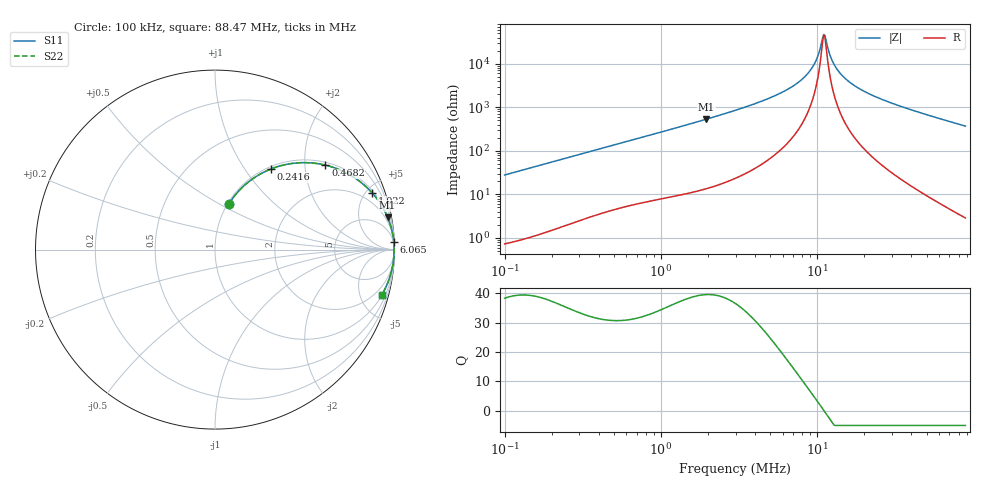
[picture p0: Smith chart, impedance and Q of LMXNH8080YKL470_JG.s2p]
! LMXNH8080YKL470_JG  S-PARAMETER MODEL  ( General Type )
! Model Generated by TAIYO YUDEN Corporation (http://www.ty-top.com)
! Version 1.0
! TAIYO YUDEN Control No. 191025NI43SB-FBB
! Copyright(c) 2019 TAIYO YUDEN CO.,LTD. All Rights Reserved.
! Product Description (link to TY-COMPAS)
! https://ds.yuden.co.jp/TYCOMPAS/or/detail?pn=LMXNH8080YKL470MJG&u=M
! Products Name : Inductors
! Characteristics :
!  Inductance : 47 uH , SRF(min) : 8.0 MHz , DC Resistance(max) : 0.182 Ohm
!  Rated Current : Saturation :1500 mA , Temp Rise : 1500 mA
!  Case Size : 8.0 x 8.0 / 0.315 x 0.315 [mm/inch] , Thickness : 4 / 0.157 [mm/inch]
!  (Conditions: Temperature = 25 degC , DC Bias Current/Voltage = 0A / 0V)
! External Node Assignments :
!  1  o---GGG---o  2
! GND o---------o GND
! Frequency Range : 0.1MHz  -  88.465963MHz  [ 402 STEP ]
# MHz S RI R 50
! Freq[MHz].  S11 Real  S11 Imag  S21 Real  S21 Imag  S12 Real  S12 Imag  S22 Real  S22 Imag
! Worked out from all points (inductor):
!   401 points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, 100 kHz to 88.47 MHz, reference 50 ohm
!   read as one part in series: L = 44.1 uH near 103.5 kHz
!   highest Q = 39.5 at 1.946 MHz (marker M1), where L = 43.4 uH
!   self-resonance near 10.98 MHz
!   S11 on the Smith chart (normalised r, x): 100 kHz: 1.01, +0.56; 241.6 kHz: 1.04, +1.33; 468.2 kHz: 1.08, +2.54; 1.022 MHz: 1.16, +5.49; 6.065 MHz: 3, +46; 88.47 MHz: 1.06, -7.38
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0.1  0.0774 0.2545  0.9226 -0.2545  0.9226 -0.2545  0.0774 0.2545
0.155432  0.1627 0.3565  0.8373 -0.3565  0.8373 -0.3565  0.1627 0.3565
0.241591  0.312 0.4494  0.688 -0.4494  0.688 -0.4494  0.312 0.4494
0.311591  0.4245 0.4794  0.5755 -0.4794  0.5755 -0.4794  0.4245 0.4794
0.468157  0.6148 0.4707  0.3852 -0.4707  0.3852 -0.4707  0.6148 0.4707
0.97089  0.8648 0.3276  0.1352 -0.3276  0.1352 -0.3276  0.8648 0.3276
1.021576  0.8759 0.3156  0.1241 -0.3156  0.1241 -0.3156  0.8759 0.3156
1.946322  0.9615 0.1801  0.0385 -0.1801  0.0385 -0.1801  0.9615 0.1801
2.974323  0.9832 0.1158  0.0168 -0.1158  0.0168 -0.1158  0.9832 0.1158
6.064564  0.9958 0.0434  0.00419 -0.0434  0.00419 -0.0434  0.9958 0.0434
7.821746  0.9972 0.024  0.00276 -0.024  0.00276 -0.024  0.9972 0.024
9.267725  0.9977 0.012  0.00227 -0.012  0.00227 -0.012  0.9977 0.012
9.918383  0.9978 0.00736  0.00216 -0.00736  0.00216 -0.00736  0.9978 0.00736
10.79632  0.9979 0.00154  0.00209 -0.00154  0.00209 -0.00154  0.9979 0.00154
11.16888  0.9979 -0.000783  0.00208 0.000783  0.00208 0.000783  0.9979 -0.000783
12.1575  0.9979 -0.0066  0.00211 0.0066  0.00211 0.0066  0.9979 -0.0066
12.57703  0.9979 -0.00893  0.00215 0.00893  0.00215 0.00893  0.9979 -0.00893
13.46002  0.9978 -0.0136  0.00224 0.0136  0.00224 0.0136  0.9978 -0.0136
14.65145  0.9976 -0.0196  0.00243 0.0196  0.00243 0.0196  0.9976 -0.0196
19.21992  0.9964 -0.0398  0.00362 0.0398  0.00362 0.0398  0.9964 -0.0398
28.8774  0.9922 -0.076  0.00784 0.076  0.00784 0.076  0.9922 -0.076
88.46596  0.9299 -0.2515  0.0701 0.2515  0.0701 0.2515  0.9299 -0.2515
